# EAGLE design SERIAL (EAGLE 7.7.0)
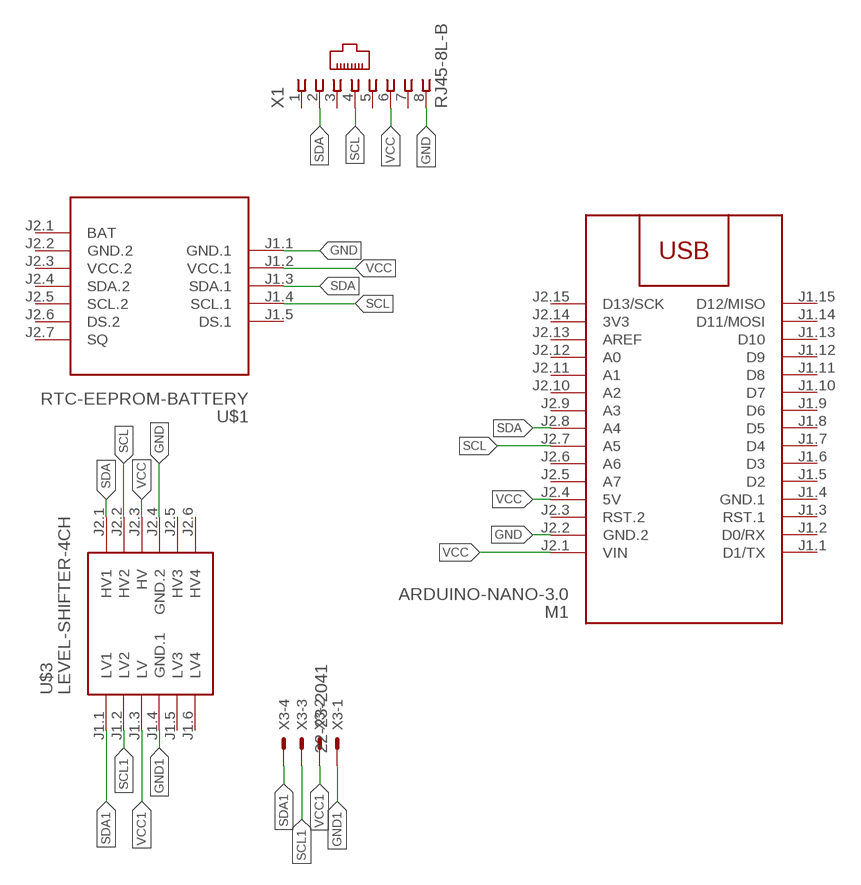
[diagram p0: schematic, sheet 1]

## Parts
M1  ARDUINO-NANO-3.0  [ARDUINO-NANO-3.0]
U$1  RTC-EEPROM-BATTERY  [RTC-EEPROM-BATTERY]
U$3  LEVEL-SHIFTER-4CH  [LEVEL-SHIFTER-4CH]
X1  RJ45-8L-B  [RJ45-NO-SHIELD]
X3  22-23-2041  [22-23-2041]

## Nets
GND: M1.J2.2(GND.2) U$1.J1.1(GND.1) U$3.J2.4(GND.2) X1.8
GND1: U$3.J1.4(GND.1) X3.1
SCL: M1.J2.7(A5) U$1.J1.4(SCL.1) U$3.J2.2(HV2) X1.4
SCL1: U$3.J1.2(LV2) X3.3
SDA: M1.J2.8(A4) U$1.J1.3(SDA.1) U$3.J2.1(HV1) X1.2
SDA1: U$3.J1.1(LV1) X3.4
VCC: M1.J2.1(VIN) M1.J2.4(5V) U$1.J1.2(VCC.1) U$3.J2.3(HV) X1.6
VCC1: U$3.J1.3(LV) X3.2
Unconnected: M1.J1.1(D1/TX) M1.J1.2(D0/RX) M1.J1.3(RST.1) M1.J1.5(D2) M1.J1.6(D3) M1.J1.7(D4) M1.J1.8(D5) M1.J1.9(D6) M1.J1.10(D7) M1.J1.11(D8) M1.J1.12(D9) M1.J1.13(D10) M1.J1.14(D11/MOSI) M1.J1.15(D12/MISO) M1.J2.3(RST.2) M1.J2.5(A7) M1.J2.6(A6) M1.J2.9(A3) M1.J2.10(A2) M1.J2.11(A1) M1.J2.12(A0) M1.J2.13(AREF) M1.J2.15(D13/SCK) U$1.J1.5(DS.1) U$1.J2.1(BAT) U$1.J2.4(SDA.2) U$1.J2.5(SCL.2) U$1.J2.6(DS.2) U$1.J2.7(SQ) U$3.J1.5(LV3) U$3.J1.6(LV4) U$3.J2.5(HV3) U$3.J2.6(HV4) X1.1 X1.3 X1.5 X1.7

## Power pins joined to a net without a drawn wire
3V3: M1.J2.14(3V3)
GND.1: M1.J1.4(GND.1)
GND.2: U$1.J2.2(GND.2)
VCC.2: U$1.J2.3(VCC.2)

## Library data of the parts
M1 = diy-modules:ARDUINO-NANO-3.0: Arduino Nano 3.0 and compatible devices More details available here: https://www.arduino.cc/en/Main/ArduinoBoardNano Click here to find device on ebay.com
U$1 = diy-modules:RTC-EEPROM-BATTERY: RTC Module with Battery and EEPROM based on DS1307 and AT24C32 chips More details available here: http://henrysbench.capnfatz.com/henrys-bench/arduino-sensors-and-input/arduino-tiny-rtc-d1307-tutorial/ Click here to find device on ebay.com
U$3 = diy-modules:LEVEL-SHIFTER-4CH: 4-Channel Bi-Directional Logic Level Converter based on BSS128 transistors Click here to find device on ebay.com
X1 = con-tycoelectronics:RJ45: CORCOM Modular RJ Jacks No Shield Source: www.tycoelectronics.com .. ENG_DS_1654001_1099_RJ_L_0507.pdf; MF: TYCO ELECTRONICS; MPN: RJ45-8L-B; OC_FARNELL: 1279843; OC_NEWARK: 52K4445
X3 = con-molex:22-23-2041: .100" (2.54mm) Center Header - 4 Pin; MF: MOLEX; MPN: 22-23-2041; OC_FARNELL: 1462920; OC_NEWARK: 38C0355

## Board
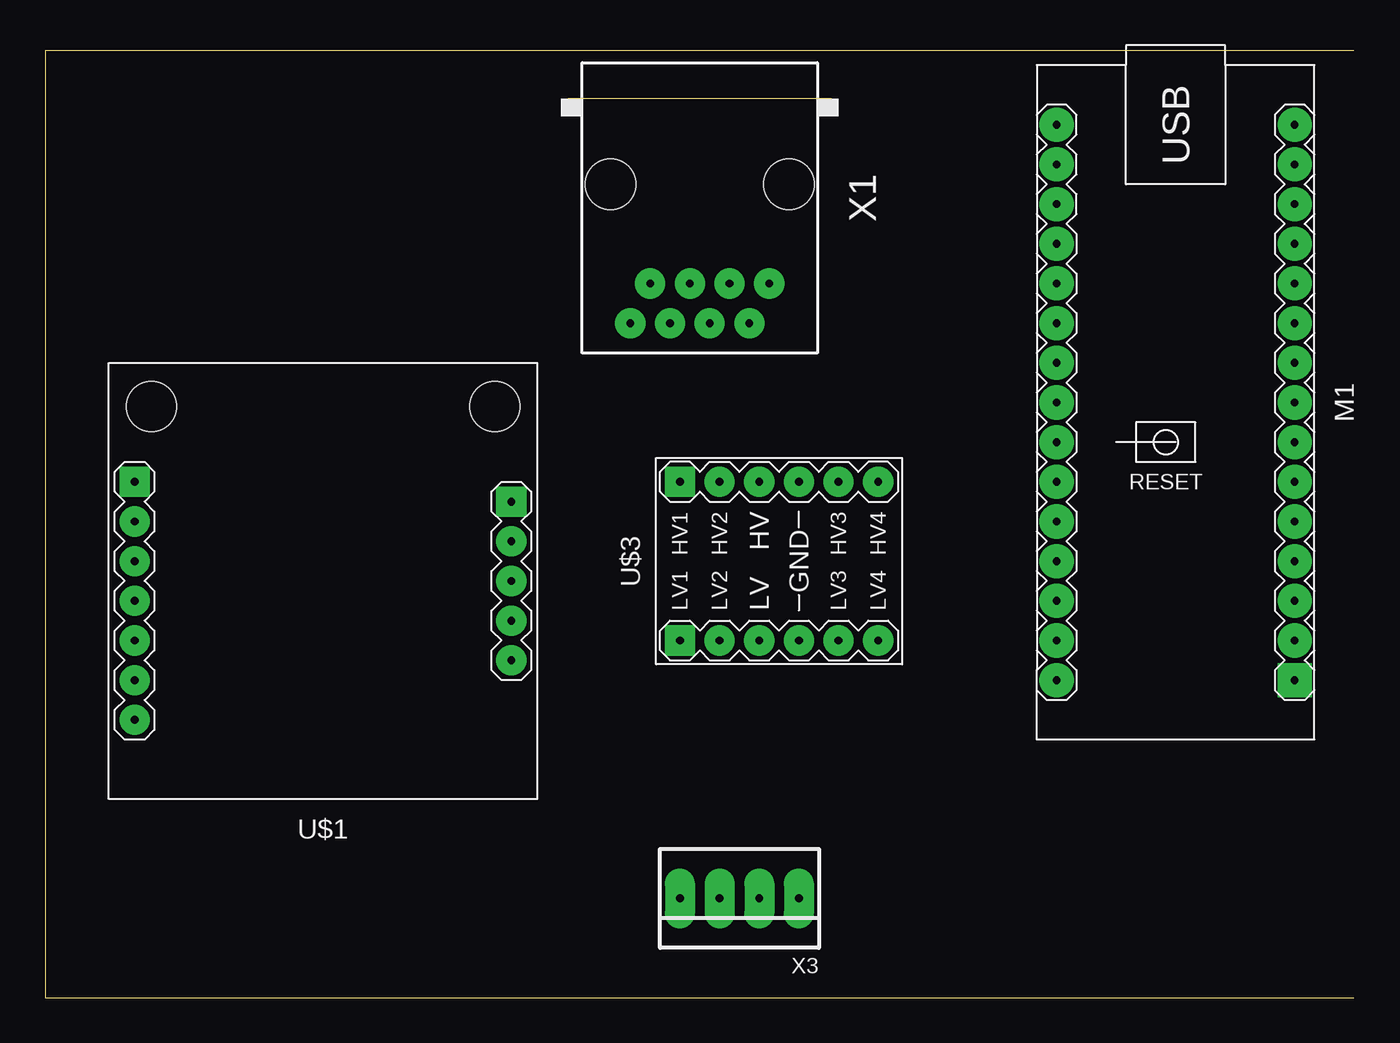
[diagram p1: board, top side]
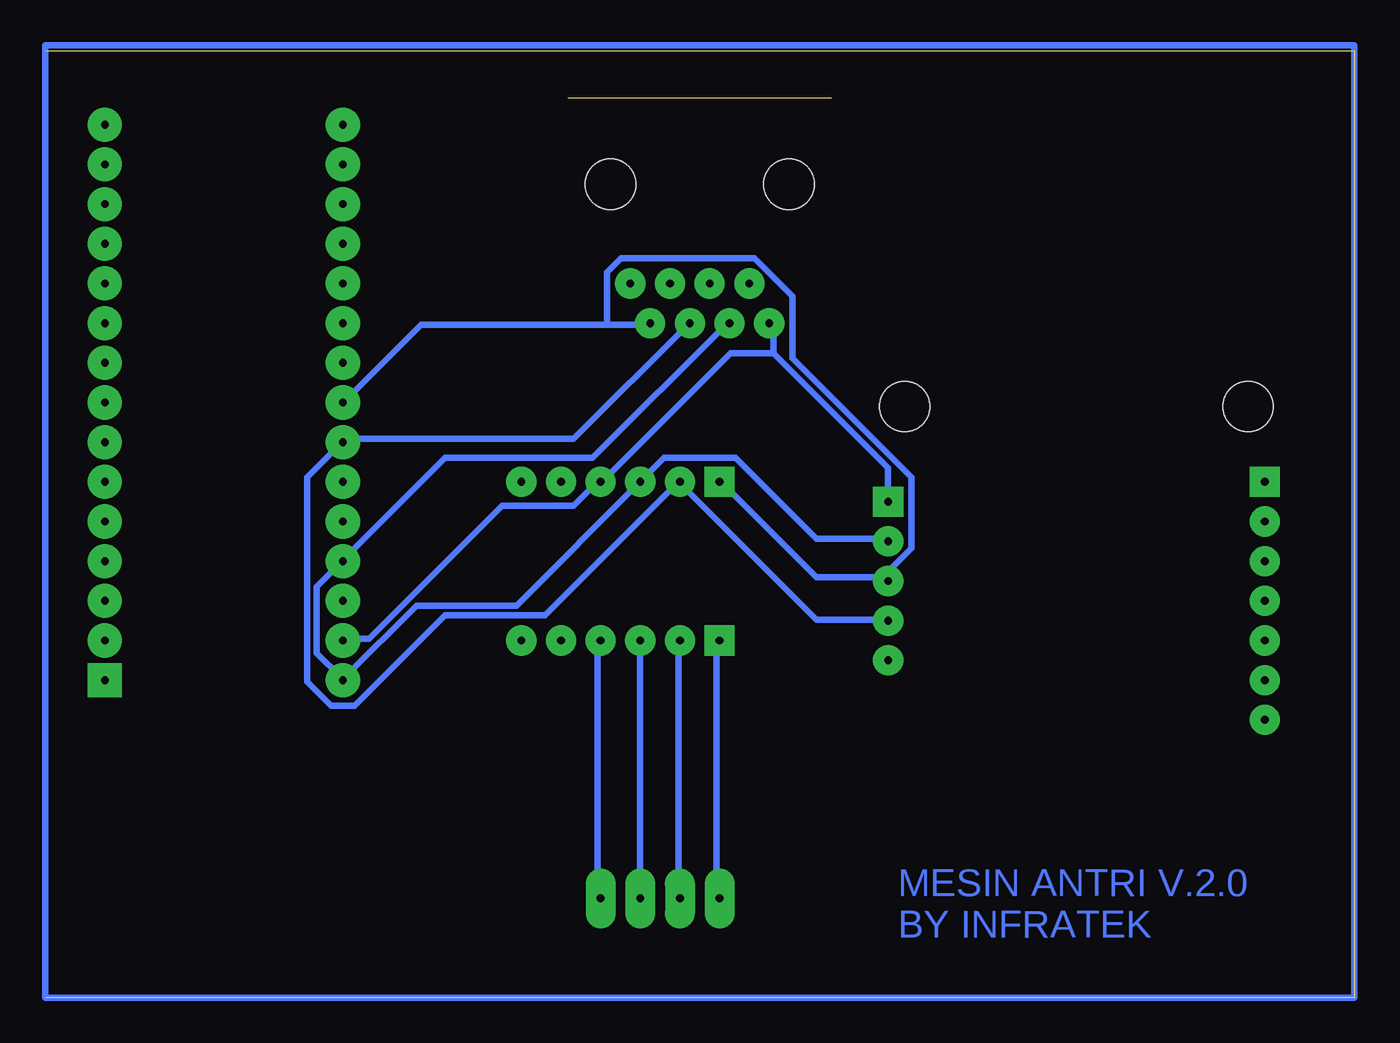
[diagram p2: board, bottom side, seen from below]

Size 83.8 x 60.63 mm. Coordinates in mm from the lower left corner, seen from the top.
Outline: 83.8,0 0,0 0,60.63 83.8,60.63
Copper layers (1*16): Top 0.035mm / dielectric 1.5mm / Bottom 0.035mm
Design rules "default *": minimum track width 16mil, minimum drill 24mil, track to track 8mil, track to pad 8mil, pad to pad 8mil, via to via 8mil, smd to smd 8mil, copper to edge 40mil, drill to drill 8mil, minimum pad ring 10mil, minimum via ring 8mil, stop-mask expansion 4mil, vias tented up to drill 0mil, thermal gap 10mil

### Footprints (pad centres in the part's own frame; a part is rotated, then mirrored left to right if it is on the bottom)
ARDUINO-NANO-3.0 = drill 0.5 pad 2.184 square: J1.1 17.78,7.62 | drill 0.5 pad 2.184: J1.2 15.24,7.62; J1.3 12.7,7.62; J1.4 10.16,7.62; J1.5 7.62,7.62; J1.6 5.08,7.62; J1.7 2.54,7.62; J1.8 0,7.62; J1.9 -2.54,7.62; J1.10 -5.08,7.62; J1.11 -7.62,7.62; J1.12 -10.16,7.62; J1.13 -12.7,7.62; J1.14 -15.24,7.62; J1.15 -17.78,7.62; J2.1 17.78,-7.62; J2.2 15.24,-7.62; J2.3 12.7,-7.62; J2.4 10.16,-7.62; J2.5 7.62,-7.62; J2.6 5.08,-7.62; J2.7 2.54,-7.62; J2.8 0,-7.62; J2.9 -2.54,-7.62; J2.10 -5.08,-7.62; J2.11 -7.62,-7.62; J2.12 -10.16,-7.62; J2.13 -12.7,-7.62; J2.14 -15.24,-7.62; J2.15 -17.78,-7.62
RTC-EEPROM-BATTERY = drill 0.5 pad 1.93 square: J1.1 -12.065,-5.08; J2.1 12.065,-6.35 | drill 0.5 pad 1.93: J1.2 -12.065,-2.54; J1.3 -12.065,0; J1.4 -12.065,2.54; J1.5 -12.065,5.08; J2.2 12.065,-3.81; J2.3 12.065,-1.27; J2.4 12.065,1.27; J2.5 12.065,3.81; J2.6 12.065,6.35; J2.7 12.065,8.89 | hole 3.2: -11,-11.176; 11,-11.176
LEVEL-SHIFTER-4CH = drill 0.5 pad 1.93 square: J1.1 -5.08,6.35; J2.1 5.08,6.35 | drill 0.5 pad 1.93: J1.2 -5.08,3.81; J1.3 -5.08,1.27; J1.4 -5.08,-1.27; J1.5 -5.08,-3.81; J1.6 -5.08,-6.35; J2.2 5.08,3.81; J2.3 5.08,1.27; J2.4 5.08,-1.27; J2.5 5.08,-3.81; J2.6 5.08,-6.35
RJ45-NO-SHIELD = drill 0.5 pad 1.93: 1 -4.445,6.35; 2 -3.175,8.89; 3 -1.905,6.35; 4 -0.635,8.89; 5 0.635,6.35; 6 1.905,8.89; 7 3.175,6.35; 8 4.445,8.89 | hole 3.251: -5.715,0; 5.715,0
22-23-2041 = drill 0.5 pad 1.93 long: 1 -3.81,0; 2 -1.27,0; 3 1.27,0; 4 3.81,0

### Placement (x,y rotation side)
M1  72.39,38.1 270 top
U$1  17.78,26.67 180 top
U$3  46.99,27.94 90 top
X1  41.91,52.07 180 top
X3  44.45,6.35 180 top

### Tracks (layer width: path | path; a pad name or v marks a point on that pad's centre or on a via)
GND
  Bottom 0.406: 37.19,41.25 29.87,33.93 29.87,31.8 U$1.J1.1 | 37.19,41.25 37.19,43.08 X1.8 | 37.19,41.25 39.93,41.25 48.16,33.02 U$3.J2.4 48.46,33.02 49.99,31.5 54.56,31.5 63.09,22.96 64.62,22.96 M1.J2.2
GND1
  Bottom 0.406: X3.1 48.46,6.5 48.46,22.66 U$3.J1.4
N$1
  Bottom 0.406: 0,60.96 0,0 83.82,0 83.82,60.96 0,60.96
SCL
  Bottom 0.406: 43.28,33.02 34.44,24.18 29.87,24.18 U$1.J1.4 | X1.4 42.67,43.08 49.99,35.76 64.62,35.76 M1.J2.7 64.92,35.46 67.06,33.32 67.06,20.22 65.53,18.69 64.01,18.69 58.22,24.49 51.82,24.49 43.28,33.02 | 43.28,33.02 U$3.J2.2
SCL1
  Bottom 0.406: X3.3 43.28,6.5 43.28,22.66 U$3.J1.2
SDA
  Bottom 0.406: U$3.J2.1 40.54,33.02 34.44,26.92 29.87,26.92 U$1.J1.3 29.57,26.92 29.57,27.53 28.35,28.75 28.35,33.32 35.97,40.95 35.97,44.91 38.41,47.35 46.94,47.35 47.85,46.43 47.85,43.08 | 47.85,43.08 59.74,43.08 64.62,38.2 M1.J2.8 | 47.85,43.08 45.11,43.08 X1.2
SDA1
  Bottom 0.406: X3.4 40.84,6.5 40.84,22.66 U$3.J1.1
VCC
  Bottom 0.406: U$1.J1.2 29.87,29.36 34.44,29.36 39.62,34.54 44.2,34.54 U$3.J2.3 53.65,25.1 60.05,25.1 64.62,20.52 M1.J2.1 64.92,20.52 66.45,22.05 66.45,26.31 64.92,27.84 M1.J2.4 64.62,28.14 58.22,34.54 48.77,34.54 40.23,43.08 X1.6
VCC1
  Bottom 0.406: U$3.J1.3 X3.2

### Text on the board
Bottom: MESIN ANTRI V.2.0 / BY INFRATEK

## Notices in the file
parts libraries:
diy-modules: Released under the Creative Commons Attribution 4.0 International License: http://creativecommons.org/licenses/by/4.0
